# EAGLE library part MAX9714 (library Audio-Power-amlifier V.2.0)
The MAX9714 mono/stereo Class D audio power amplifiers provide Class AB amplifier performance with Class D efficiency, conserving board space and eliminating the need for a bulky heatsink. Using a Class D architecture, these devices deliver up to 6W while offering greater than 85% efficiency. Proprietary and protected modulation and switching schemes render the traditional Class D output filter unnecessary.
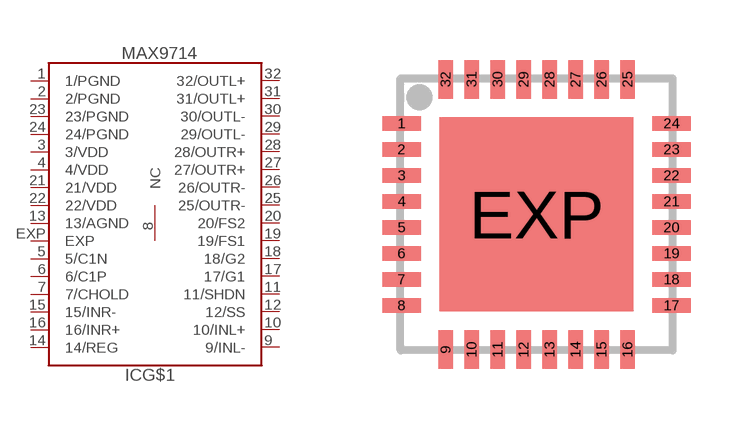
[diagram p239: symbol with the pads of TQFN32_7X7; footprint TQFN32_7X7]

Designator prefix IC; gates G$1=MAX9714 G$2=NC

## MAX9714  [TQFN32_7X7]
1  G$1:1/PGND  pwr
2  G$1:2/PGND  pwr
3  G$1:3/VDD  pwr
4  G$1:4/VDD  pwr
5  G$1:5/C1N
6  G$1:6/C1P
7  G$1:7/CHOLD
8  G$2:NC  nc
9  G$1:9/INL-  in
10  G$1:10/INL+  in
11  G$1:11/SHDN
12  G$1:12/SS
13  G$1:13/AGND  pwr
14  G$1:14/REG  out
15  G$1:15/INR-  in
16  G$1:16/INR+  in
17  G$1:17/G1  in
18  G$1:18/G2  in
19  G$1:19/FS1  in
20  G$1:20/FS2  in
21  G$1:21/VDD  pwr
22  G$1:22/VDD  pwr
23  G$1:23/PGND  pwr
24  G$1:24/PGND  pwr
25  G$1:25/OUTR-  out
26  G$1:26/OUTR-  out
27  G$1:27/OUTR+  out
28  G$1:28/OUTR+  out
29  G$1:29/OUTL-  out
30  G$1:30/OUTL-  out
31  G$1:31/OUTL+  out
32  G$1:32/OUTL+  out
EXP  G$1:EXP  pwr

## Footprint TQFN32_7X7 (pad centres in mm)
TQFN 7x7 mm Source: www.maxim-ic.com/packages .. 90-0125.pdf
smd 0.965 x 0.366: 1 -3.378,2.275; 2 -3.378,1.625; 3 -3.378,0.975; 4 -3.378,0.325; 5 -3.378,-0.325; 6 -3.378,-0.975; 7 -3.378,-1.625; 8 -3.378,-2.275; 17 3.378,-2.275; 18 3.378,-1.625; 19 3.378,-0.975; 20 3.378,-0.325; 21 3.378,0.325; 22 3.378,0.975; 23 3.378,1.625; 24 3.378,2.275
smd 0.366 x 0.965: 9 -2.275,-3.378; 10 -1.625,-3.378; 11 -0.975,-3.378; 12 -0.325,-3.378; 13 0.325,-3.378; 14 0.975,-3.378; 15 1.625,-3.378; 16 2.275,-3.378; 25 2.275,3.378; 26 1.625,3.378; 27 0.975,3.378; 28 0.325,3.378; 29 -0.325,3.378; 30 -0.975,3.378; 31 -1.625,3.378; 32 -2.275,3.378
smd 4.851 x 4.851: EXP 0,0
